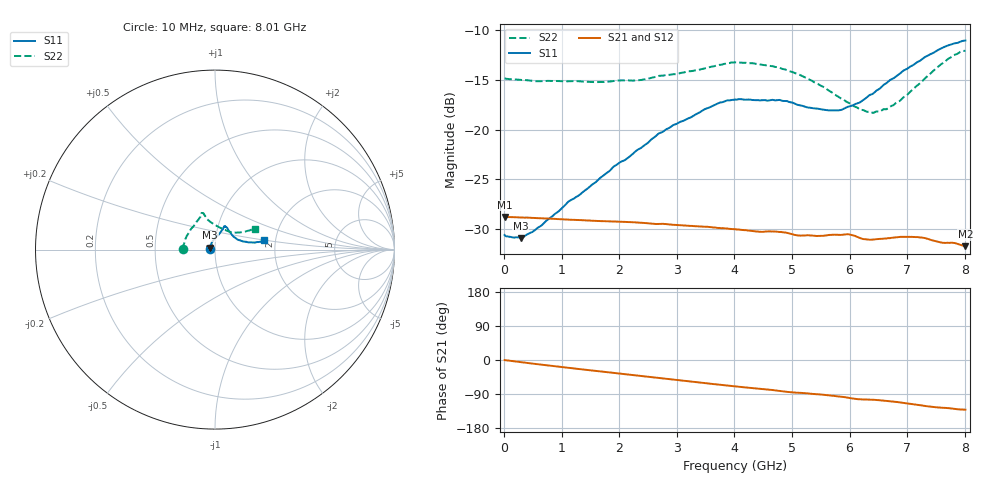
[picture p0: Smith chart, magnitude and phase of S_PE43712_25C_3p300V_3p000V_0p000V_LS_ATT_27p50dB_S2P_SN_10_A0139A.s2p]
! DEVICE ID: PE43712
! File Path: z:\PE43713\PE43713_CHAR_NOM_04292014\AMB\3p300\LS_ATT_27p50dB\PE43713_AMB_3p300V_3p000V_0p000V_LS_ATT_27p50dB_S2P_SN_10_A0139A.s2p
! Serial: 10
! Lot: A0139A
! Temp: 25C
! VDD: 3.300
! VSS: 0.000
! Control_Hi: 3.000
! Control_Lo: 0.000
! Attenuation Step: 27.50dB
! Port 1: RF1
! Port 2: RF2
! ThroughPath:1-2
! IDD: 0.0001453327
! ISS: -9.47e-008
#  Hz  S  RI  R  50
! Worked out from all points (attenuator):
!   801 points, 10 MHz to 8.01 GHz, reference 50 ohm
!   highest |S21| = -28.76 dB at 10 MHz (marker M1); lowest = -31.7 dB at 8.01 GHz (marker M2)
!   lowest |S11| = -30.9 dB at 290 MHz (marker M3), VSWR 1.06, Z = 47.4 + j1.03 ohm
!   |S11| at or under -10 dB: start of sweep to end of sweep
!   |S22| runs from -18.3 to -12.1 dB; largest |S21 - S12| = 0.00015
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1e7  -0.0296 0.000777  0.0365 -0.00015  0.0365 -0.000141  -0.1806 0.00116
2.9e8  -0.0265 0.0109  0.0361 -0.00358  0.0361 -0.00359  -0.1764 0.0189
6.4e8  -0.0235 0.0231  0.0351 -0.00758  0.0351 -0.00757  -0.1703 0.0395
1.12e9  -0.0179 0.0398  0.0331 -0.0125  0.0331 -0.0125  -0.1615 0.0672
1.35e9  -0.0133 0.0463  0.032 -0.0146  0.032 -0.0147  -0.1555 0.0785
2.3e9  0.0135 0.0774  0.0259 -0.0224  0.0258 -0.0224  -0.1203 0.129
2.68e9  0.0267 0.0915  0.0228 -0.0247  0.0228 -0.0247  -0.1036 0.1542
3.5e9  0.0458 0.1187  0.0158 -0.0285  0.0157 -0.0285  -0.079 0.1872
3.74e9  0.0496 0.1271  0.0135 -0.0292  0.0135 -0.0292  -0.0763 0.197
4.01e9  0.0534 0.131  0.0111 -0.0297  0.0111 -0.0297  -0.0751 0.204
4.76e9  0.0638 0.1257  0.00469 -0.0304  0.00476 -0.0304  -0.06 0.1962
5.35e9  0.0804 0.0998  0.000318 -0.0294  0.000346 -0.0294  -0.044 0.1699
5.87e9  0.1047 0.0702  -0.00371 -0.0295  -0.00368 -0.0295  -0.00721 0.1423
5.99e9  0.113 0.0657  -0.00522 -0.0294  -0.00514 -0.0294  0.00375 0.1361
6.17e9  0.1242 0.0568  -0.00676 -0.0278  -0.00668 -0.0278  0.0219 0.1246
6.31e9  0.1366 0.0522  -0.00703 -0.0273  -0.00695 -0.0272  0.0388 0.1166
6.42e9  0.1445 0.049  -0.00728 -0.0272  -0.00722 -0.0271  0.0513 0.1103
6.68e9  0.1699 0.0436  -0.00902 -0.0271  -0.00898 -0.027  0.0823 0.0993
7.17e9  0.2139 0.0399  -0.0136 -0.0255  -0.0136 -0.0255  0.1359 0.0958
7.55e9  0.2484 0.0433  -0.0158 -0.0223  -0.0158 -0.0223  0.1805 0.104
7.81e9  0.2659 0.0481  -0.0169 -0.0211  -0.0169 -0.0211  0.2072 0.1128
8.01e9  0.2751 0.0521  -0.0171 -0.0196  -0.017 -0.0197  0.2203 0.1162
